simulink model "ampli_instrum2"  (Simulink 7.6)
settings: Solver=ode15s  StartTime=0.0  StopTime=0.004  RelTol=1e-3
StopFcn:
  | close all, clc
  | load signaux_es.mat
  | plot(x(1,:),x(2,:),x(1,:),x(3,:),x(1,:),x(4,:))
  | title('Amplificateur d''instrumentation')
  | xlabel('temps')
  | grid
libraries: fl_lib x22, nesl_utility x5, simulink x1

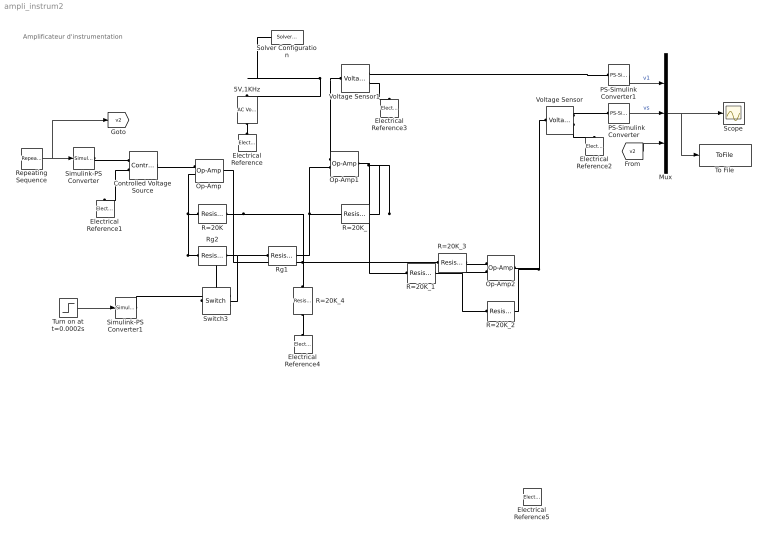
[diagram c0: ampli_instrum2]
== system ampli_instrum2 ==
  note: Amplificateur d'instrumentation
  5V,1KHz : fl_lib/Electrical/Electrical Sources/AC Voltage Source  DialogController=NetworkEngine.DynNeDlgSource  SystemSampleTime=-1  amp=0.5 V  shift=0 rad  omega=1000 Hz  i_Log=off  v_Log=off  LocalVarNames=|current|voltage|power  LocalVarDescs=|Current (A)|Voltage (V)|Power (W)  LocalVarLogging=[0 0 0]
  Controlled Voltage Source : fl_lib/Electrical/Electrical Sources/Controlled Voltage Source  DialogController=NetworkEngine.DynNeDlgSource  SystemSampleTime=-1  i_Log=off  v_Log=off  LocalVarNames=|i|v  LocalVarDescs=|i|v  LocalVarLogging=[0 0]
  Electrical Reference{,1..5} (6 alike) : fl_lib/Electrical/Electrical Elements/Electrical Reference  DialogController=NetworkEngine.DynNeDlgSource  SystemSampleTime=-1  i_Log=off  LocalVarNames=|i  LocalVarDescs=|i  LocalVarLogging=[]
  Mux : Mux  Inputs=3
  Op-Amp : fl_lib/Electrical/Electrical Elements/Op-Amp  DialogController=NetworkEngine.DynNeDlgSource  SystemSampleTime=-1  i1_Log=off  v1_Log=off  outI_Log=off  LocalVarNames=|i1|v1|outI  LocalVarDescs=|i1|v1|outI  LocalVarLogging=[]
  Op-Amp1 : fl_lib/Electrical/Electrical Elements/Op-Amp  DialogController=NetworkEngine.DynNeDlgSource  SystemSampleTime=-1  i1_Log=off  v1_Log=off  outI_Log=off  LocalVarNames=|i1|v1|outI  LocalVarDescs=|i1|v1|outI  LocalVarLogging=[]
  Op-Amp2 : fl_lib/Electrical/Electrical Elements/Op-Amp  DialogController=NetworkEngine.DynNeDlgSource  SystemSampleTime=-1  i1_Log=off  v1_Log=off  outI_Log=off  LocalVarNames=|i1|v1|outI  LocalVarDescs=|i1|v1|outI  LocalVarLogging=[]
  PS-Simulink Converter : nesl_utility/PS-Simulink Converter  DialogController=NetworkEngine.DynNeUtilDlgSource  SystemSampleTime=-1  PhysicalDomain=network_engine_domain  LeftPortType=input  RightPortType=output  SubClassName=ps_output  Unit=1  AffineConversion=off
  PS-Simulink Converter1 : nesl_utility/PS-Simulink Converter  DialogController=NetworkEngine.DynNeUtilDlgSource  SystemSampleTime=-1  PhysicalDomain=network_engine_domain  LeftPortType=input  RightPortType=output  SubClassName=ps_output  Unit=1  AffineConversion=off
  R=20K : fl_lib/Electrical/Electrical Elements/Resistor  DialogController=NetworkEngine.DynNeDlgSource  SystemSampleTime=-1  R=20e3 Ohm  i_Log=off  v_Log=off  LocalVarNames=|current|voltage|power  LocalVarDescs=|Resistor current (A)|Voltage across resistor (V)|Power (W)  LocalVarLogging=[0 0 0]
  R=20K_{,1..4} (5 alike) : fl_lib/Electrical/Electrical Elements/Resistor  DialogController=NetworkEngine.DynNeDlgSource  SystemSampleTime=-1  R=20e3 Ohm  i_Log=off  v_Log=off  LocalVarNames=|current|voltage|power  LocalVarDescs=|Resistor current (A)|Voltage across resistor (V)|Power (W)  LocalVarLogging=[0 0 0]
  Repeating Sequence : simulink/Sources/Repeating Sequence  SystemSampleTime=-1  rep_seq_t=[0 0.001 0.002]  rep_seq_y=[0 1 0]
  Rg1 : fl_lib/Electrical/Electrical Elements/Resistor  DialogController=NetworkEngine.DynNeDlgSource  SystemSampleTime=-1  R=20e3 Ohm  i_Log=off  v_Log=off  LocalVarNames=|current|voltage|power  LocalVarDescs=|Resistor current (A)|Voltage across resistor (V)|Power (W)  LocalVarLogging=[0 0 0]
  Rg2 : fl_lib/Electrical/Electrical Elements/Resistor  DialogController=NetworkEngine.DynNeDlgSource  SystemSampleTime=-1  R=20 kOhm  i_Log=off  v_Log=off  LocalVarNames=|current|voltage|power  LocalVarDescs=|Resistor current (A)|Voltage across resistor (V)|Power (W)  LocalVarLogging=[0 0 0]
  Scope : Scope
  Simulink-PS Converter : nesl_utility/Simulink-PS Converter  DialogController=NetworkEngine.DynNeUtilDlgSource  SystemSampleTime=-1  PhysicalDomain=network_engine_domain  LeftPortType=input  RightPortType=output  SubClassName=ps_input  Unit=1  AffineConversion=off  InputFilterTimeConstant=.001  UdotUserProvided=0
  Simulink-PS Converter1 : nesl_utility/Simulink-PS Converter  DialogController=NetworkEngine.DynNeUtilDlgSource  SystemSampleTime=-1  PhysicalDomain=network_engine_domain  LeftPortType=input  RightPortType=output  SubClassName=ps_input  Unit=1  AffineConversion=off  InputFilterTimeConstant=.001  UdotUserProvided=0
  Solver Configuration : nesl_utility/Solver Configuration  DialogController=NetworkEngine.DynNeUtilDlgSource  SystemSampleTime=-1  PhysicalDomain=network_engine_domain  LeftPortType=input  RightPortType=generic  SubClassName=solver  Accelerate=off  Profile=off  ResidualTolerance=1e-9  MaxNonlinIter=12  MaxModeIter=2  DoFixedCost=off  UseLocalSampling=off  DoDC=off  LinearAlgebra=Sparse  LocalSolverSampleTime=.001  LocalSolverChoice=NE_BACKWARD_EULER_ADVANCER  UseLocalSolver=off
  Switch3 : fl_lib/Electrical/Electrical Elements/Switch  DialogController=NetworkEngine.DynNeDlgSource  SystemSampleTime=-1  R_closed=0.01 Ohm  G_open=1e-08 1/Ohm  Threshold=0  i_Log=off  v_Log=off  LocalVarNames=|current|voltage|power  LocalVarDescs=|Current (A)|Voltage (V)|Power (W)  LocalVarLogging=[0 0 0]
  To File : ToFile  Filename=signaux_es  MatrixName=x
  Turn on at t=0.0002s : Step  Time=0.002
  Voltage Sensor : fl_lib/Electrical/Electrical Sensors/Voltage Sensor  DialogController=NetworkEngine.DynNeDlgSource  SystemSampleTime=-1  i1_Log=off  v1_Log=off  LocalVarNames=|i1|v1  LocalVarDescs=|i1|v1  LocalVarLogging=[]
  Voltage Sensor1 : fl_lib/Electrical/Electrical Sensors/Voltage Sensor  DialogController=NetworkEngine.DynNeDlgSource  SystemSampleTime=-1  i1_Log=off  v1_Log=off  LocalVarNames=|i1|v1  LocalVarDescs=|i1|v1  LocalVarLogging=[]
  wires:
  PS-Simulink Converter1/1 -> Mux/1  "v1"
  PS-Simulink Converter/1 -> Mux/2  "vs"
  Mux/1 -> Scope/1, To File/1
  [v2] -> Mux/3
  Turn on at t=0.0002s/1 -> Simulink-PS Converter1/1
  Repeating Sequence/1 -> [v2], Simulink-PS Converter/1
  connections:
  Rg2/RConn1 -- Op-Amp/LConn2 -- R=20K/LConn1 -- Switch3/RConn2
  Op-Amp/RConn1 -- R=20K/RConn1 -- R=20K_3/LConn1 -- R=20K_4/LConn1
  Rg1/RConn1 -- R=20K_/LConn1 -- Op-Amp1/LConn2
  Voltage Sensor/RConn1 -- PS-Simulink Converter/LConn1
  Voltage Sensor/RConn2 -- Electrical Reference2/LConn1
  Voltage Sensor1/RConn1 -- PS-Simulink Converter1/LConn1
  Voltage Sensor1/RConn2 -- Electrical Reference3/LConn1
  5V,1KHz/RConn1 -- Electrical Reference/LConn1
  Op-Amp1/RConn1 -- R=20K_/RConn1 -- R=20K_1/LConn1
  Op-Amp1/LConn1 -- Solver Configuration/RConn1 -- 5V,1KHz/LConn1 -- Voltage Sensor1/LConn1
  R=20K_1/RConn1 -- Op-Amp2/LConn2 -- R=20K_2/LConn1
  R=20K_3/RConn1 -- Op-Amp2/LConn1
  R=20K_4/RConn1 -- Electrical Reference4/LConn1
  Rg2/LConn1 -- Rg1/LConn1 -- Switch3/LConn1
  Simulink-PS Converter1/RConn1 -- Switch3/RConn1
  Simulink-PS Converter/RConn1 -- Controlled Voltage Source/RConn1
  Controlled Voltage Source/LConn1 -- Op-Amp/LConn1
  Controlled Voltage Source/RConn2 -- Electrical Reference1/LConn1
  Voltage Sensor/LConn1 -- Op-Amp2/RConn1 -- R=20K_2/RConn1
  Electrical Reference5/LConn1 -- ?
